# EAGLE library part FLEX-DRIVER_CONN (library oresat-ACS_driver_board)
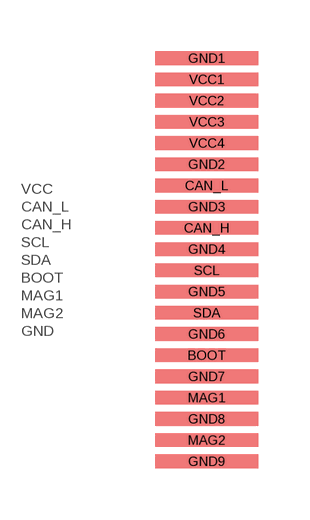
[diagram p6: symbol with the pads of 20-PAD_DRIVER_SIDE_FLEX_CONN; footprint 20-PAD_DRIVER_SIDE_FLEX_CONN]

Designator prefix -

## FLEX-DRIVER_CONN  [20-PAD_DRIVER_SIDE_FLEX_CONN]
BOOT  BOOT
CAN_H  CAN_H
CAN_L  CAN_L
GND1  GND
GND2  GND
GND3  GND
GND4  GND
GND5  GND
GND6  GND
GND7  GND
GND8  GND
GND9  GND
MAG1  MAG1
MAG2  MAG2
SCL  SCL
SDA  SDA
VCC1  VCC
VCC2  VCC
VCC3  VCC
VCC4  VCC

## Footprint 20-PAD_DRIVER_SIDE_FLEX_CONN (pad centres in mm)
smd 3 x 0.4: BOOT 0,-2.79; CAN_H 0,0.93; CAN_L 0,2.17; GND1 0,5.89; GND2 0,2.79; GND3 0,1.55; GND4 0,0.31; GND5 0,-0.93; GND6 0,-2.17; GND7 0,-3.41; GND8 0,-4.65; GND9 0,-5.89; MAG1 0,-4.03; MAG2 0,-5.27; SCL 0,-0.31; SDA 0,-1.55; VCC1 0,5.27; VCC2 0,4.65; VCC3 0,4.03; VCC4 0,3.41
